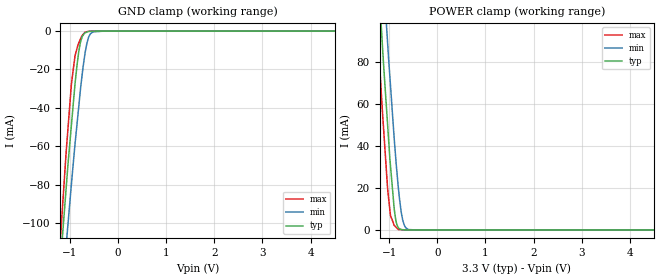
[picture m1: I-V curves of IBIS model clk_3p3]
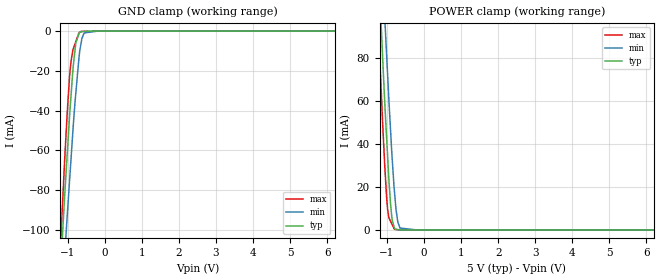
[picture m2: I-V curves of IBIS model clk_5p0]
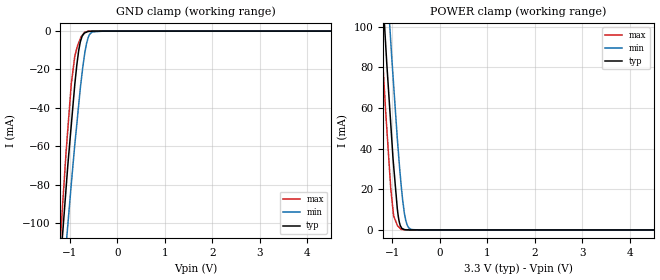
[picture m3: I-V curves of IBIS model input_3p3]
|Texas Instruments Incorporated
|12-Bit, 6 MSPS ADC Quad Ch. (Config.), DSP/uP IF, Integ. 16x FIFO, Channel
|AutoScan, Low Power
| Marketing part#   Digital Voltage Range   Package-type   #pins
| THS1206CDA   3.0V - 5.25V   TSSOP   32
| THS1206CDAG4   3.0V - 5.25V   TSSOP   32
| THS1206CDAR   3.0V - 5.25V   TSSOP   32
| THS1206CDARG4   3.0V - 5.25V   TSSOP   32
| THS1206IDA   3.0V - 5.25V   TSSOP   32
| THS1206IDAG4   3.0V - 5.25V   TSSOP   32
| THS1206IDAR   3.0V - 5.25V   TSSOP   32
| THS1206IDARG4   3.0V - 5.25V   TSSOP   32
| THS1206QDA   3.0V - 5.25V   TSSOP   32
| THS1206QDAR   3.0V - 5.25V   TSSOP   32
[IBIS Ver]   3.2
[File name]   ths1206.ibs
|SIMDE Ver   V3.0 - 201101 - Build 457
[File Rev]   1.0
[Date]   12/19/2011
[Source]
| Texas Instruments Incorporated.
| Analog-eLab Design Center, HPA
| 12500 TI Blvd
| Dallas, TX -75243
| e-mail: elab_scm_ibis@list.ti.com
[Notes]   Revision History:
| Rev 1.0: 12/19/2011
| - Initial version of the model
| - Model generated from simulations in TISPICE
| - Model matched to SPICE simulation
| - C_comp although listed in numerical order of value are
|   obtained from varying PVT conditions. For PVT conditions for
|   each specific value refer the buffer description under
|   respective [Model]. IBIS model user is responsible for using
|   appropriate C_comp to simulate for Signal Integrity.
| - Model names with a trailing _3p3 contains the model for
|   3.3V [3.0V and 3.6V]. Model names with a trailing _5 contains
|   the model for 5.0V [4.75V and 5.25V].
[Disclaimer]
| This model is designed as an aid for customers of Texas Instruments.
| TI and its licensors and suppliers make no warranties, either expressed
| or implied, with respect to this  model, including the warranties of
| merchantability or fitness for a particular purpose. The model is
| provided solely on an "as is" basis. The entire risk as to its quality
| and performance is with the customer.
[Copyright]
 (C) Copyright 2011 Texas Instruments Incorporated.All rights reserved.
|   THS1206
[Component]   THS1206
[Manufacturer]   TI
[Package]   |32 TSSOP   -  DA package
|   typ   min   max
R_pkg   0.10991   0.09834   0.12955
L_pkg   3.57749nH   2.80072nH   5.32816nH
C_pkg   0.77494pF   0.66520pF   0.90891pF
[Pin]  signal_name   model_name   R_pin   L_pin   C_pin
1   D0   DB   0.12840   5.19909nH  0.89675pF
2   D1   DB   0.11651   4.20090nH  0.84289pF
3   D2   DB   0.11428   3.56834nH  0.78147pF
4   D3   DB   0.11374   3.49051nH  0.77966pF
5   D4   DB   0.10789   3.24123nH  0.76928pF
6   D5   DB   0.10444   3.09241nH  0.71111pF
7   BVDD   POWER   0.10061   2.91471nH  0.68417pF
8   BGND   GND   0.09766   2.78878nH  0.66001pF
9   D6   DB   0.09895   2.81728nH  0.68213pF
10   D7   DB   0.10101   2.92173nH  0.68129pF
11   D8   DB   0.10425   3.08864nH  0.70997pF
12   D9   DB   0.10842   3.25741nH  0.76938pF
13   D10/RA0   DB   0.11268   3.46954nH  0.78054pF
14   D11/RA1   DB   0.11429   3.57685nH  0.78213pF
15   CONV_CLK(_CONVST)   CLK   0.11657   4.21210nH  0.84643pF
16   DATA_AV   DATA   0.12817   5.20011nH  0.89944pF
17   DGND   GND   0.12632   5.17483nH  0.89879pF
18   DVDD   POWER   0.11565   4.19931nH  0.84772pF
19   _RD   INPUT   0.10913   3.49538nH  0.78998pF
20   _WR(R/_W)   INPUT   0.10850   3.40770nH  0.78028pF
21   CS1   INPUT   0.10483   3.19492nH  0.76783pF
22   _CS0   INPUT   0.10259   3.06553nH  0.70865pF
23   AVDD   POWER   0.10101   2.92801nH  0.67919pF
24   AGND   GND   0.06484   2.51469nH  0.70709pF
25   REFM   TERM   0.09834   2.80072nH  0.66520pF
26   REFP   TERM   0.10013   2.90513nH  0.68890pF
27   REFOUT   TERM   0.10445   3.10254nH  0.71388pF
28   REFIN   TERM   0.10306   3.16116nH  0.76027pF
29   BINM   TERM   0.10333   3.31687nH  0.73212pF
30   BINP   TERM   0.11077   3.58492nH  0.82081pF
31   AINM   TERM   0.11331   4.31556nH  0.87902pF
32   AINP   TERM   0.12955   5.32816nH  0.90891pF
1000   thermal_pad   NC   0.00003   0.00172nH  3.26032pF
|   Model Selectors
[Model Selector] CLK
clk_3p3  3.3V digital input
clk_5p0  5.0V digital input
[Model Selector] INPUT
input_3p3  3.3V digital input
input_5p0  5.0V digital input
[Model Selector] DATA
data_3p3  3.3V digital output
data_5p0  5.0V digital output
[Model Selector] DB
db_3p3  3.3V digital I/O
db_5p0  5.0V digital I/O
[Model Selector] TERM
term_3-3V  3.3V nominal termination
term_5-0V  5.0V nominal termination
[Model] term_3-3V
Model_type Terminator
C_comp   1.0e-20F  1.0e-20F  1.0e-20F
|   typ   min   max
[Voltage Range]   3.3V   3.0V   3.6V
[POWER Clamp Reference]   3.3V   3.0V   3.6V
[GND Clamp Reference]   0V   0V   0V
|Ambient Temperature   25   125   -55
|Junction Temperature
[Temperature Range]   43   145   -55
[Model] term_5-0V
Model_type Terminator
C_comp   1.0e-20F  1.0e-20F  1.0e-20F
|   typ   min   max
[Voltage Range]   5.0V   4.75V   5.25V
[POWER Clamp Reference]   5.0V   4.75V   5.25V
[GND Clamp Reference]   0V   0V   0V
|Ambient Temperature   25   125   -55
|Junction Temperature
[Temperature Range]   43   145   -55
| Models and submodels in the file (10): clk_3p3 (Input), clk_5p0 (Input), input_3p3 (Input), input_5p0 (Input), data_3p3 (Output), data_5p0 (Output), db_3p3 (I/O), db_5p0 (I/O), term_3-3V (Terminator), term_5-0V (Terminator)
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|   clk_3p3 Model
[Model]   clk_3p3
Model_type   Input
Vinl = 0.6
Vinh = 2
|   typ   min   max
|   (nom PVT)   (fast PVT)   (slow PVT)
 C_comp   1.052e-12   1.043e-12   1.060e-12
| Where nom  PVT is Nominal Process, 3.3V, 43C
|   Fast PVT is Strong Process,  3.6V, -55C
|   Slow PVT is Weak Process,   3V, 145C
[Voltage Range]   3.3   3   3.6
|Ambient Temperature   25   125   -55
|Junction Temperature
[Temperature Range]   43   145   -55
[Power Clamp Reference]   3.3   3   3.6
[GND Clamp Reference]   0   0   0
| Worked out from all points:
|   GND clamp passes 1 mA (typ) near -0.69 V on its own axis
|   POWER clamp passes 1 mA (typ) near -0.81 V on its own axis
[GND Clamp]
|   Voltage   I(typ)   I(min)   I(max)
-3.3V     -930.8mA   -899mA     -1.009A
-1.241V   -134mA     -161.3mA   -123.5mA
-1.084V   -82.61mA   -112.5mA   -63.84mA
-1.043V   -69.28mA   -100.4mA   -50.5mA
-972mV    -48.99mA   -79.71mA   -27.55mA
-896.4mV  -27.37mA   -58.68mA   -12.8mA
-818.4mV  -10.59mA   -39.07mA   -6.201mA
-782.1mV  -5.643mA   -29.95mA   -4.006mA
-684mV    -903.4uA   -10.83mA   -543.2uA
-579mV    -122.4uA   -1.472mA   -55.45uA
-285mV    -10.1uA    -1.059uA   -32.66nA
6.6V      0A         0A         0A
[POWER Clamp]
|   Voltage   I(typ)   I(min)   I(max)
-3.3V     976.8mA    997mA      970.3mA
-1.31V    151.5mA    190.7mA    122.1mA
-1.17V    98.33mA    137.9mA    66.95mA
-1.141V   87.43mA    127.3mA    56.13mA
-1.037V   50.93mA    89.86mA    20.52mA
-975.6mV  30.84mA    69.16mA    6.972mA
-897.6mV  10.21mA    43.61mA    2.234mA
-854.7mV  3.735mA    31.2mA     1.194mA
-813.6mV  1.246mA    20.71mA    241.2uA
-723mV    87.08uA    4.975mA    129.3uA
-591mV    13.97uA    182.9uA    14.83uA
6.6V      0A         0A         0A
|   clk_5p0 Model
[Model]   clk_5p0
Model_type   Input
Vinl = 0.6
Vinh = 2.6
|   typ   min   max
|   (nom PVT)   (fast PVT)   (slow PVT)
C_comp   9.597e-13   9.486e-13   9.672e-13
| Where nom  PVT is Nominal Process, 5V, 43C
|   Fast PVT is Strong Process,  5.25V, -55C
|   Slow PVT is Weak Process,   4.75V, 145C
[Voltage Range]   5   4.75   5.25
|Ambient Temperature   25   125   -55
|Junction Temperature
[Temperature Range]   43   145   -55
[Power Clamp Reference]   5   4.75   5.25
[GND Clamp Reference]   0   0   0
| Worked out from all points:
|   GND clamp passes 1 mA (typ) near -0.69 V on its own axis
|   POWER clamp passes 1 mA (typ) near -0.80 V on its own axis
[GND Clamp]
|   Voltage   I(typ)   I(min)   I(max)
-5V       -1.63A     -1.558A    -1.765A
-1.306V   -156.5mA   -182mA     -149mA
-1.08V    -80.95mA   -111.4mA   -62.58mA
-1.021V   -63.13mA   -93.97mA   -42.58mA
-913.5mV  -32.25mA   -64mA      -15.06mA
-855mV    -17.62mA   -47.73mA   -8.966mA
-785mV    -5.956mA   -31.17mA   -5.31mA
-698.3mV  -1.195mA   -13.09mA   -779.1uA
-640.5mV  -317.8uA   -5.762mA   -155.4uA
-560.5mV  -201.6uA   -951.6uA   -136uA
-190mV    0A         -86.58nA   -46.1uA
10V       0A         0A         0A
[POWER Clamp]
|   Voltage   I(typ)   I(min)   I(max)
-5V       1.713A     1.721A     1.716A
-1.306V   150.8mA    189.6mA    122.6mA
-1.118V   80.04mA    119.5mA    49.44mA
-1.045V   53.51mA    92.83mA    24.89mA
-981.8mV  33.3mA     71.13mA    9.228mA
-905mV    12.03mA    46.28mA    4.044mA
-860mV    4.422mA    32.77mA    2.402mA
-803.3mV  1.109mA    18.55mA    330.8uA
-707.7mV  136.1uA    3.593mA    152uA
-650.8mV  37.52uA    898.8uA    45.25uA
-190mV    0A         0A         7.728uA
10V       0A         0A         0A
|   input_3p3 Model
[Model]   input_3p3
Model_type   Input
Vinl = 0.6
Vinh = 2
|   typ   min   max
|   (nom PVT)   (fast PVT)   (slow PVT)
C_comp   1.052e-12   1.043e-12   1.060e-12
| Where nom  PVT is Nominal Process, 3.3V, 43C
|   Fast PVT is Strong Process,  3.6V, -55C
|   Slow PVT is Weak Process,   3V, 145C
[Voltage Range]   3.3   3   3.6
|Ambient Temperature   25   125   -55
|Junction Temperature
[Temperature Range]   43   145   -55
[Power Clamp Reference]   3.3   3   3.6
[GND Clamp Reference]   0   0   0
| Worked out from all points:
|   GND clamp passes 1 mA (typ) near -0.69 V on its own axis
|   POWER clamp passes 1 mA (typ) near -0.81 V on its own axis
[GND Clamp]
|   Voltage   I(typ)   I(min)   I(max)
-3.3V     -930.8mA   -899mA     -1.009A
-1.241V   -134mA     -161.3mA   -123.5mA
-1.084V   -82.61mA   -112.5mA   -63.84mA
-1.043V   -69.28mA   -100.4mA   -50.5mA
-972mV    -48.99mA   -79.71mA   -27.55mA
-896.4mV  -27.37mA   -58.68mA   -12.8mA
-818.4mV  -10.59mA   -39.07mA   -6.201mA
-782.1mV  -5.643mA   -29.95mA   -4.006mA
-684mV    -903.4uA   -10.83mA   -543.2uA
-579mV    -122.4uA   -1.472mA   -55.45uA
-285mV    -10.1uA    -1.059uA   -32.66nA
6.6V      0A         0A         0A
[POWER Clamp]
|   Voltage   I(typ)   I(min)   I(max)
-3.3V     1.015A     1.036A     1.007A
-1.307V   155.5mA    196.5mA    124.9mA
-1.167V   100.7mA    141.8mA    67.91mA
-1.115V   80.48mA    122.5mA    48.72mA
-1.037V   52.57mA    93.12mA    20.93mA
-975.6mV  31.74mA    71.52mA    7.004mA
-897.6mV  10.4mA     44.96mA    2.234mA
-854.7mV  3.771mA    32.08mA    1.194mA
-813.6mV  1.252mA    21.21mA    241.2uA
-723mV    87.08uA    5.027mA    129.3uA
-591mV    13.97uA    183uA      14.83uA
6.6V      0A         0A         0A
